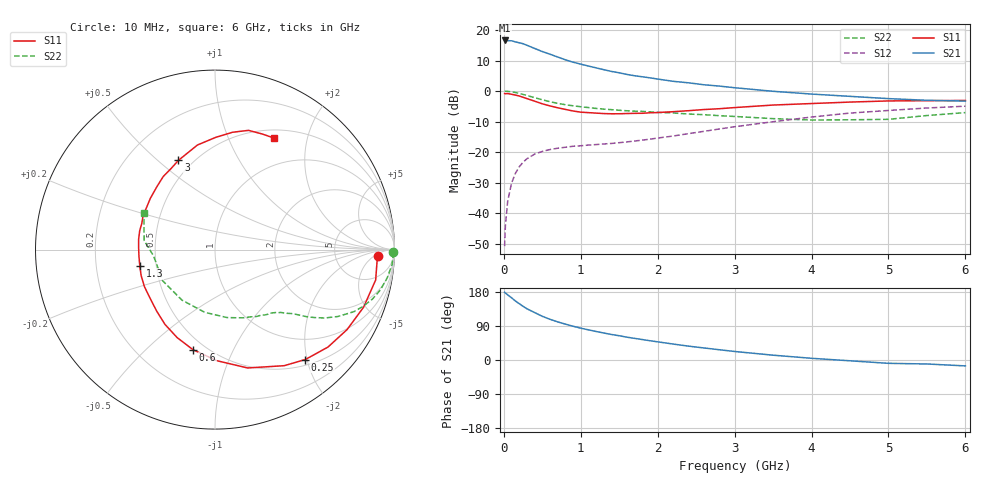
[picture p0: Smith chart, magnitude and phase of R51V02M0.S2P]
! SIEMENS Small Signal Semiconductors
! BFR183
! Si NPN RF Bipolar Junction Transistor in SOT23
! VCE = 1 V  IC = 2 mA
! Common Emitter S-Parameters:  May  1996
# GHz  S  MA  R  50
!  f  S11  S21  S12  S22
! GHz  MAG  ANG  MAG  ANG  MAG  ANG  MAG  ANG
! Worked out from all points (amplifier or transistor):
!   36 points, 10 MHz to 6 GHz, reference 50 ohm
!   highest |S21| = 16.6 dB at 10 MHz (marker M1)
!   |S21| within 3 dB of that: start of sweep to 438.3 MHz
!   unconditionally stable (mu >= 1): 1.35 GHz to 3.053 GHz
!   at 250 MHz: K = 0.23, MSG = 19.4 dB, |S12| = -23.3 dB
!   at 1.4 GHz: K = 1.03, MAG = 10.8 dB, |S12| = -17.1 dB
!   at 6 GHz: K = 0.95, MSG = 0.8 dB, |S12| = -4.9 dB
!   S11 on the Smith chart (normalised r, x): 10 MHz: 18, -7; 250 MHz: 0.60, -1.97; 600 MHz: 0.43, -0.71; 1.3 GHz: 0.40, -0.09; 3 GHz: 0.42, +0.59; 6 GHz: 0.60, +1.48
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0.01  0.9094 -2.2  6.737 178.8  0.0029 88.0  0.9945 -0.9
0.02  0.9053 -4.2  6.696 176.7  0.0062 84.4  0.993 -2.0
0.05  0.911 -10.7  6.678 172.0  0.0158 84.8  0.9898 -4.8
0.1  0.8878 -21.2  6.653 164.2  0.0311 78.2  0.9725 -9.3
0.15  0.8603 -31.2  6.386 155.8  0.045 72.3  0.9484 -13.7
0.25  0.7926 -50.6  5.954 141.6  0.0684 62.7  0.8822 -21.1
0.3  0.753 -59.2  5.621 135.2  0.0782 58.6  0.8472 -24.1
0.4  0.684 -74.6  4.99 125.2  0.0929 52.3  0.7806 -28.5
0.5  0.6192 -89.0  4.435 115.3  0.1031 47.3  0.7212 -31.9
0.6  0.5715 -102.3  4.012 107.4  0.1106 44.0  0.6702 -34.4
0.7  0.5337 -113.3  3.611 100.6  0.1161 41.6  0.6309 -36.3
0.8  0.5013 -123.8  3.253 94.6  0.1205 39.8  0.5978 -37.7
1  0.4519 -143.2  2.759 84.0  0.1275 38.3  0.5541 -40.0
1.1  0.4441 -152.3  2.568 79.6  0.1308 38.4  0.5369 -41.4
1.3  0.4286 -167.8  2.239 71.2  0.1365 39.4  0.5067 -43.7
1.6  0.4295 172.2  1.872 60.2  0.1475 41.9  0.4762 -47.8
2.2  0.4599 141.5  1.446 42.1  0.1839 47.1  0.4384 -58.3
3  0.5373 112.3  1.135 22.5  0.261 47.2  0.3844 -80.0
3.5  0.591 99.5  0.992 12.7  0.3156 43.3  0.3541 -99.3
4.5  0.661 81.5  0.82 -2.1  0.4368 31.0  0.3391 -148.9
5.5  0.6961 67.5  0.707 -10.5  0.5287 17.0  0.3981 172.7
6  0.7025 62.3  0.686 -15.6  0.5663 8.2  0.4447 152.9
